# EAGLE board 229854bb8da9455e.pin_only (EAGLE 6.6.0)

Size 27.94 x 29.21 mm. Coordinates in mm from the lower left corner, seen from the top.
Outline: 2.54,29.21 25.4,29.21 arc-90 27.94,26.67 27.94,2.54 arc-90 25.4,0 2.54,0 arc-90 0,2.54 0,26.67 arc-90 2.54,29.21
Copper layers (1*16): Top 0.035mm / dielectric 1.5mm / Bottom 0.035mm
Design rules "adafruit": minimum track width 8mil, minimum drill 15.5mil, track to track 8mil, track to pad 8mil, pad to pad 8mil, via to via 8mil, smd to smd 8mil, copper to edge 10mil, drill to drill 8mil, minimum pad ring 10mil, minimum via ring 8mil, stop-mask expansion 2mil, vias tented up to drill 20mil, thermal gap 10mil
Holes 3.2 mm at 2.54,22.86 25.4,22.86
tRestrict: area 10.3,13.2 to 10.6,13.3

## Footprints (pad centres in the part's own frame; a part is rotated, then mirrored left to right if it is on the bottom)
0805-NO = smd 1.3 x 1.5: 1 -0.95,0; 2 0.95,0
_0402 = smd 0.6 x 0.6: 1 -0.508,0; 2 0.508,0
_0402MP = smd 0.5 x 0.5: 1 -0.508,0; 2 0.508,0
_0603 = smd 0.9 x 0.8: 1 -0.762,0; 2 0.762,0
0805 = smd 1.3 x 1.5: 1 -0.95,0; 2 0.95,0
FIDUCIAL_1MM = smd 1 x 1: 1 0,0
1X10_ROUND70 = drill 1 pad 1.778 square: 1 -11.43,0 | drill 1 pad 1.778: 2 -8.89,0; 3 -6.35,0; 4 -3.81,0; 5 -1.27,0; 6 1.27,0; 7 3.81,0; 8 6.35,0; 9 8.89,0; 10 11.43,0
_0805MP = smd 1.2 x 1.3: 1 -1.016,0; 2 1.016,0
QFN32_5MM = smd 0.8 x 0.25: 1 -2.5,1.75; 2 -2.5,1.25; 3 -2.5,0.75; 4 -2.5,0.25; 5 -2.5,-0.25; 6 -2.5,-0.75; 7 -2.5,-1.25; 8 -2.5,-1.75; 17 2.5,-1.75; 18 2.5,-1.25; 19 2.5,-0.75; 20 2.5,-0.25; 21 2.5,0.25; 22 2.5,0.75; 23 2.5,1.25; 24 2.5,1.75 | smd 0.25 x 0.8: 9 -1.75,-2.5; 10 -1.25,-2.5; 11 -0.75,-2.5; 12 -0.25,-2.5; 13 0.25,-2.5; 14 0.75,-2.5; 15 1.25,-2.5; 16 1.75,-2.5; 25 1.75,2.5; 26 1.25,2.5; 27 0.75,2.5; 28 0.25,2.5; 29 -0.25,2.5; 30 -0.75,2.5; 31 -1.25,2.5; 32 -1.75,2.5 | smd 3.5 x 3.5: 33 0,0
SOT23-5 = smd 0.55 x 1.2: 1 -0.95,-1.3; 2 0,-1.3; 3 0.95,-1.3; 4 0.95,1.3; 5 -0.95,1.3
TSSOP16 = smd 0.305 x 0.991: 1 -2.275,-2.918; 2 -1.625,-2.918; 3 -0.975,-2.918; 4 -0.325,-2.918; 5 0.325,-2.918; 6 0.975,-2.918; 7 1.625,-2.918; 8 2.275,-2.918; 9 2.275,2.918; 10 1.625,2.918; 11 0.975,2.918; 12 0.325,2.918; 13 -0.325,2.918; 14 -0.975,2.918; 15 -1.625,2.918; 16 -2.275,2.918
ANT_PCB_2.4GHZ_NRF8001_1.6MM_1OZ = smd 1.27 x 1.27: FEED 0,0; TESTPOINT -8.169,17.605
CRYSTAL_3.2X2.5 = smd 1.4 x 1.2: 1 -1.1,-0.8; 2 1.1,0.8; GND1 -1.1,0.8; GND2 1.1,-0.8
CRYSTAL_8X3.8 = smd 1.3 x 1.9: P$1 -2.75,-1.6; P$2 2.75,-1.6; P$3 2.75,1.6; P$4 -2.75,1.6

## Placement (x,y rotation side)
C1  15pF  [0805-NO]  2.45,12.55 180 top
C2  15pF  [0805-NO]  2.78,19.12 0 top
C3  2.2nF  [_0402]  15.75,19.33 0 top
C4  0.1µF  [0805-NO]  2.38,8.74 180 top
C5  1.8pF  [_0402MP]  8.35,18.2 0 top
C6  1.2pF  [_0402MP]  6.55,18.2 0 top
C7  1µF  [0805-NO]  2.38,10.64 180 top
C8  1nF  [_0603]  7.88,13.45 180 top
C9  10µF  [0805-NO]  5.8,5.93 0 top
C10  0.1uF  [0805-NO]  8.5,7 270 top
C11  33nF  [0805-NO]  10.27,7 270 top
C12  0.1µF  [0805-NO]  18.02,11.1 0 top
C13  15pF  [0805-NO]  23.14,7.24 90 top
C14  15pF  [0805-NO]  12.07,7 90 top
C15  1.5pF  [_0402MP]  6.55,19.4 0 top
C16  10µF  [0805-NO]  25.82,5.66 180 top
C17  10µF  [0805-NO]  26.48,13 90 top
FB1  MMZ1608B121C  [0805]  5.25,8.86 90 top
FID1  FIDUCIAL""  [FIDUCIAL_1MM]  16.98,7.04 270 top
FID2  FIDUCIAL""  [FIDUCIAL_1MM]  26.61,18.88 270 top
FID3  FIDUCIAL""  [FIDUCIAL_1MM]  2.13,27.24 270 top
JP1  [1X10_ROUND70]  13.97,2.54 0 top
L1  8.2nH  [_0402]  12.45,18.2 180 top
L2  5.6nH  [_0402]  13.45,19.33 0 top
L3  3.9nH  [_0402]  10.33,18.2 180 top
L4  10µH  [_0603]  7.89,10.15 180 top
L5  15nH  [_0603]  7.89,11.79 0 top
R1  22K  [_0805MP]  7.98,16.49 180 top
R2  10K  [0805-NO]  2.27,6.84 0 top
U1  nRF8001  [QFN32_5MM]  12.92,14.23 90 top
U2  MIC5225-3.3v  [SOT23-5]  25.87,8.68 0 top
U3  74HC4050D  [TSSOP16]  21.27,14.67 270 top
U$22  [ADAFRUIT_TEXT_20MM]  24.8,12.01 0 bottom
U$28  [ANT_PCB_2.4GHZ_NRF8001_1.6MM_1OZ]  7.43,18.52 270 top
Y1  16MHz  [CRYSTAL_3.2X2.5]  2.55,15.64 270 top
Y2  FC-255 32.7680K-A3  [CRYSTAL_8X3.8]  17.9,6.91 0 top

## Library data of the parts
C1-C15 FB1 L1-L5 R1 U1-U3 U$22 U$28 Y1 Y2 = microbuilder
C16 C17 JP1 R2 = microbuilder; AUTHOR: K. Townsend
FID1 FID2 = microbuilder; BOM: EXCLUDE
FID3 = microbuilder; AUTHOR: K. Townsend; BOM: EXCLUDE

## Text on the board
tPlace: nRF8001 | Bluetooth LE | v1.1 | SCK | MOSI | RDY | RST | GND | MISO | REQ | ACT | 3Vo | VIN
bPlace: VIN: 3.3-5V | LOGIC: 5V Safe

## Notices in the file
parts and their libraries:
microbuilder: This work is placed in the public domain, and may be freely used for commercial and non-commercial work with the following conditions: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
